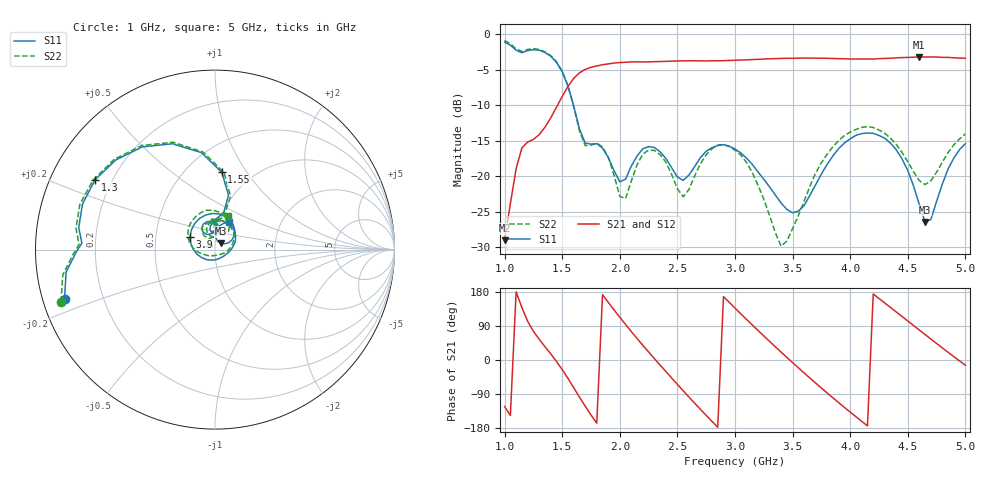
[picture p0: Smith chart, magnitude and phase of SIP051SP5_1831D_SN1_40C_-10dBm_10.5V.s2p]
# GHz  S  dB  R  50
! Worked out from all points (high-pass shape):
!   81 points, 1 GHz to 5 GHz, reference 50 ohm
!   highest |S21| = -3.18 dB at 4.6 GHz (marker M1); lowest = -29.0 dB at 1 GHz (marker M2)
!   |S21| within 3 dB of the highest: 1.602 GHz to end of sweep
!   lowest |S11| = -26.5 dB at 4.65 GHz (marker M3), VSWR 1.10, Z = 53.2 + j3.71 ohm
!   |S11| at or under -10 dB: 1.598 GHz to end of sweep
!   |S22| runs from -29.9 to -0.9 dB; largest |S21 - S12| = 0.0028
!   S11 on the Smith chart (normalised r, x): 1 GHz: 0.06, -0.16; 1.3 GHz: 0.14, +0.26; 1.55 GHz: 0.73, +0.78; 3.9 GHz: 0.75, +0.11; 5 GHz: 1.11, +0.35
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1  -1.09 -162.0  -29.05 -122.7  -28.98 -123.3  -0.86 -161.3
1.15  -2.59 177.2  -16.02 138.3  -16.01 138.1  -2.41 177.9
1.3  -2.23 149.8  -14.14 54.7  -14.14 54.7  -2.14 150.2
1.45  -3.94 111.9  -10.28 -3.7  -10.28 -3.6  -3.85 111.4
1.55  -7.28 85.0  -7.34 -48.5  -7.32 -48.6  -7.29 83.3
1.7  -15.34 87.5  -4.93 -122.1  -4.94 -122.2  -15.69 88.6
1.85  -16.04 91.7  -4.29 172.4  -4.29 172.4  -15.86 89.0
2.05  -20.42 118.0  -3.93 93.7  -3.94 93.8  -23.15 116.3
2.2  -16.14 115.2  -3.89 38.7  -3.88 38.8  -16.90 120.7
2.35  -16.57 91.1  -3.83 -13.5  -3.84 -13.5  -16.96 92.7
2.6  -19.84 102.4  -3.73 -97.7  -3.73 -97.6  -21.89 108.9
2.8  -15.98 86.3  -3.73 -161.8  -3.73 -161.8  -16.12 97.5
3  -16.16 49.5  -3.65 137.0  -3.64 137.1  -16.34 54.5
3.2  -19.41 13.3  -3.52 77.9  -3.51 77.8  -21.29 7.1
3.4  -23.78 -27.8  -3.39 20.8  -3.39 20.8  -29.87 -71.9
3.7  -21.20 -149.2  -3.35 -60.9  -3.36 -60.9  -19.56 -175.7
3.9  -16.10 152.7  -3.43 -112.4  -3.43 -112.6  -14.98 148.1
4.15  -13.91 94.4  -3.47 -173.8  -3.48 -173.7  -13.00 102.0
4.35  -15.34 53.4  -3.37 138.5  -3.37 138.5  -14.63 69.1
4.6  -23.99 30.6  -3.18 79.1  -3.19 79.1  -20.63 61.8
4.65  -26.46 47.1  -3.19 67.2  -3.18 67.3  -21.18 74.1
5  -15.42 63.1  -3.37 -14.0  -3.37 -13.8  -14.04 68.9
